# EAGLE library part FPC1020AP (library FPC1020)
FPC1020AP Fingerprint Sensor LGA Package
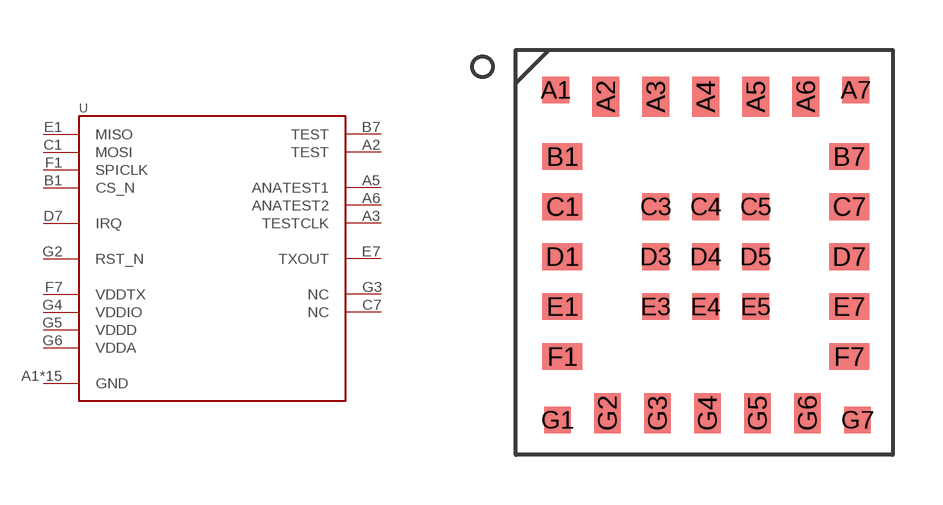
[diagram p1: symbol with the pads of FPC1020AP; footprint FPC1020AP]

Designator prefix -

## FPC1020AP  [FPC1020AP]
A1  GND  pwr
A2  TEST
A3  TESTCLK
A4  GND  pwr
A5  ANATEST1
A6  ANATEST2
A7  GND  pwr
B1  CS_N  in
B7  TEST
C1  MOSI
C3  GND  pwr
C4  GND  pwr
C5  GND  pwr
C7  NC  nc
D1  GND  pwr
D3  GND  pwr
D4  GND  pwr
D5  GND  pwr
D7  IRQ  out
E1  MISO
E3  GND  pwr
E4  GND  pwr
E5  GND  pwr
E7  TXOUT  out
F1  SPICLK  in
F7  VDDTX  pwr
G1  GND  pwr
G2  RST_N  in
G3  NC  nc
G4  VDDIO  pwr
G5  VDDD  pwr
G6  VDDA  pwr
G7  GND  pwr

## Footprint FPC1020AP (pad centres in mm)
FPC1020AP - TOUCH FINGERPRINT SENSOR LGA PACKAGE
smd 0.8 x 0.8: A1 1.2,-1.2; A7 10.2,-1.2; C3 4.2,-4.7; C4 5.7,-4.7; C5 7.2,-4.7; D3 4.2,-6.2; D4 5.7,-6.2; D5 7.2,-6.2; E3 4.2,-7.7; E4 5.7,-7.7; E5 7.2,-7.7; G1 1.25,-11.1; G7 10.25,-11.1
smd 0.8 x 1.2: A2 2.7,-1.4; A3 4.2,-1.4; A4 5.7,-1.4; A5 7.2,-1.4; A6 8.7,-1.4; G2 2.75,-10.9; G3 4.25,-10.9; G4 5.75,-10.9; G5 7.25,-10.9; G6 8.75,-10.9
smd 1.2 x 0.8: B1 1.4,-3.2; B7 10,-3.2; C1 1.4,-4.7; C7 10,-4.7; D1 1.4,-6.2; D7 10,-6.2; E1 1.4,-7.7; E7 10,-7.7; F1 1.4,-9.2; F7 10,-9.2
